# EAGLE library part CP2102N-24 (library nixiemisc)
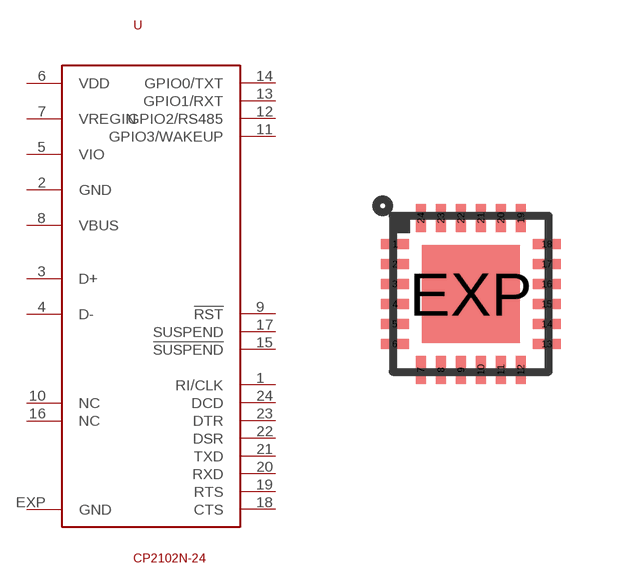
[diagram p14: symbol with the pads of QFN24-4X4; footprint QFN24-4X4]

Designator prefix U

## CP2102N-24  [QFN24-4X4]
1  RI/CLK
2  GND  pwr
3  D+  in
4  D-  in
5  VIO  pwr
6  VDD  pwr
7  VREGIN  pwr
8  VBUS  pwr
9  !RST!
10  NC  nc
11  GPIO3/WAKEUP
12  GPIO2/RS485
13  GPIO1/RXT
14  GPIO0/TXT
15  !SUSPEND!  out
16  NC  nc
17  SUSPEND  out
18  CTS  in
19  RTS  out
20  RXD  in
21  TXD  out
22  DSR  in
23  DTR  out
24  DCD  in
EXP  GND  pwr

## Footprint QFN24-4X4 (pad centres in mm)
UF Package 24-Lead (4mm × 4mm) Plastic QFN Source: http://cds.linear.com/docs/Datasheet/5598f.pdf
smd 0.7 x 0.25: 1 -1.9,1.25; 2 -1.9,0.75; 3 -1.9,0.25; 4 -1.9,-0.25; 5 -1.9,-0.75; 6 -1.9,-1.25; 13 1.9,-1.25; 14 1.9,-0.75; 15 1.9,-0.25; 16 1.9,0.25; 17 1.9,0.75; 18 1.9,1.25
smd 0.25 x 0.7: 7 -1.25,-1.9; 8 -0.75,-1.9; 9 -0.25,-1.9; 10 0.25,-1.9; 11 0.75,-1.9; 12 1.25,-1.9; 19 1.25,1.9; 20 0.75,1.9; 21 0.25,1.9; 22 -0.25,1.9; 23 -0.75,1.9; 24 -1.25,1.9
smd 2.45 x 2.45: EXP 0,0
